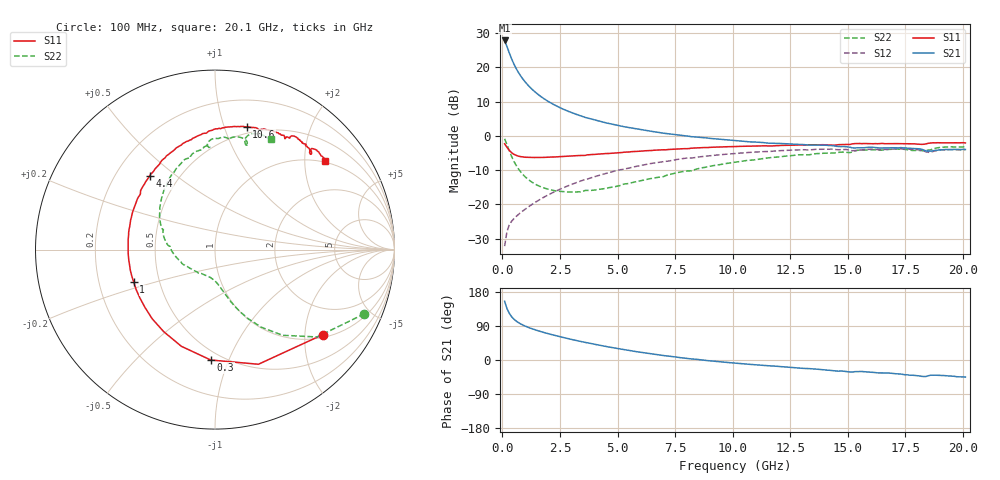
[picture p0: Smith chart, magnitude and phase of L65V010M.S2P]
!  Infineon Technologies AG
! BFR380L3 , PF131585-7, No.6, Th 09.10.01, soldered on pcb-board, measured with PP GSG850
!  Vce=5.0 V,  Ic=10.0 mA
! Common Emitter S-Parameters:  15. November 2001
#  GHz  S  MA  R  50
! f  S11  S21  S12  S22
! GHz  Mag  Ang  Mag  Ang  Mag  Ang  Mag  Ang
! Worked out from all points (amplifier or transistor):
!   201 points, 100 MHz to 20.1 GHz, reference 50 ohm
!   highest |S21| = 27.8 dB at 100 MHz (marker M1)
!   |S21| within 3 dB of that: start of sweep to 268.7 MHz
!   unconditionally stable (mu >= 1): 1.875 GHz to 4.467 GHz
!   at 3.4 GHz: K = 1.03, MAG = 8.4 dB, |S12| = -13.2 dB
!   at 10.1 GHz: K = 0.94, MSG = 1.9 dB, |S12| = -5.1 dB
!   at 20.1 GHz: K = 0.99, MSG = 0.0 dB, |S12| = -4.0 dB
!   S11 on the Smith chart (normalised r, x): 100 MHz: 1.08, -2.47; 300 MHz: 0.44, -0.86; 1 GHz: 0.36, -0.17; 4.4 GHz: 0.34, +0.40; 10.6 GHz: 0.44, +1.19; 20.1 GHz: 0.96, +2.51
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0.1  0.7652 -38.2  24.51 155.0  0.02471 70.6  0.9059 -23.3
0.2  0.683 -69.3  20.11 136.2  0.03988 59.6  0.7483 -40.6
0.3  0.6155 -92.2  16.23 123.4  0.05034 53.2  0.6079 -51.7
0.4  0.5704 -109.2  13.34 114.5  0.0568 50.1  0.5034 -59.2
0.5  0.5391 -122.0  11.19 107.9  0.06205 49.4  0.4275 -64.3
0.6  0.5206 -132.3  9.589 102.9  0.06694 49.4  0.372 -68.1
0.7  0.5059 -140.5  8.38 98.7  0.07165 49.8  0.3299 -71.1
0.8  0.4978 -147.2  7.432 95.1  0.07635 50.5  0.2975 -73.5
1  0.4878 -158.1  6.054 89.3  0.08593 52.2  0.2517 -77.4
1.2  0.4855 -166.3  5.106 84.4  0.09578 53.7  0.2214 -80.8
1.4  0.4838 -173.4  4.417 80.2  0.1061 55.0  0.2004 -83.9
1.6  0.4841 -179.2  3.894 76.3  0.1167 56.0  0.1854 -87.0
1.9  0.4872 173.3  3.318 71.0  0.1331 56.7  0.1704 -91.7
2.6  0.4993 158.9  2.484 60.1  0.1726 56.8  0.1544 -104.3
3.5  0.5175 143.8  1.905 47.6  0.2257 54.3  0.1554 -120.8
4.4  0.5488 131.6  1.577 37.0  0.2784 50.5  0.1696 -140.2
6.8  0.623 104.8  1.121 13.3  0.4136 36.3  0.2499 177.1
10.1  0.6982 78.8  0.8538 -8.3  0.5535 14.6  0.4131 136.1
10.6  0.707 75.5  0.8261 -11.0  0.57 11.3  0.4371 130.6
13.5  0.7381 60.9  0.7382 -23.5  0.631 -7.1  0.5417 104.1
16.8  0.7707 48.3  0.6698 -34.6  0.6383 -23.9  0.6353 80.7
20.1  0.7891 38.9  0.6327 -45.1  0.6303 -38.0  0.6919 63.3
